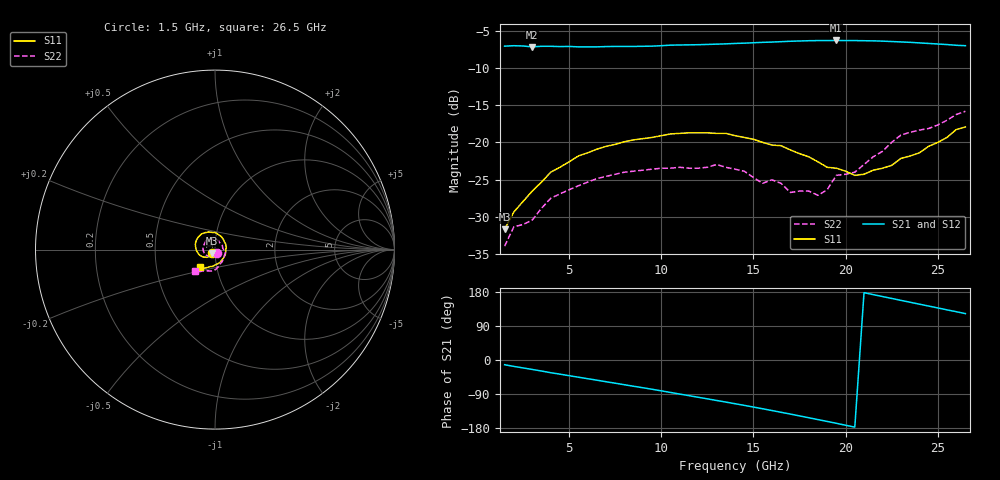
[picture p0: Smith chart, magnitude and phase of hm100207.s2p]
! HMMC-1002
! S-PARAMETERS at 7 dB attenuation setting. LAST UPDATED  07-06-99
# GHZ  S  MA  R  50
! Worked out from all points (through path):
!   51 points, 1.5 GHz to 26.5 GHz, reference 50 ohm
!   highest |S21| = -6.27 dB at 19.5 GHz (marker M1); lowest = -7.1 dB at 3 GHz (marker M2)
!   group delay of S21, straight-line fit = 24.9 ps
!   lowest |S11| = -31.7 dB at 1.5 GHz (marker M3), VSWR 1.05, Z = 48.2 - j1.82 ohm
!   |S11| at or under -10 dB: start of sweep to end of sweep
!   |S22| runs from -34.0 to -15.8 dB; largest |S21 - S12| = 0.0071
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1.5  0.026 -133.5  0.445 -12.5  0.442 -12.9  0.02 -62.8
2  0.034 -124.6  0.448 -16.9  0.446 -17.3  0.027 -70.5
3  0.047 -133.3  0.44 -24.9  0.441 -25.3  0.03 -103.0
4  0.063 -136.5  0.444 -33.5  0.443 -33.7  0.042 -108.9
6  0.085 -155.5  0.44 -49.3  0.44 -49.5  0.054 -139.9
8  0.101 -173.7  0.443 -65.3  0.442 -65.4  0.063 -161.9
10  0.111 169.1  0.448 -81.4  0.448 -81.5  0.067 175.9
13  0.115 136.8  0.459 -106.8  0.458 -106.8  0.071 136.1
14  0.111 124.4  0.464 -115.4  0.462 -115.3  0.066 124.2
15.5  0.1 103.6  0.472 -128.7  0.472 -128.7  0.053 93.2
16  0.096 97.8  0.474 -133.3  0.474 -133.2  0.056 81.7
16.5  0.095 90.0  0.477 -138.0  0.476 -137.9  0.053 66.5
17  0.089 81.1  0.48 -142.7  0.478 -142.6  0.046 60.4
18  0.08 63.5  0.484 -152.3  0.483 -152.2  0.047 29.2
18.5  0.074 51.2  0.485 -157.3  0.484 -157.1  0.044 10.0
19  0.068 40.1  0.485 -162.1  0.485 -161.9  0.048 0.3
19.5  0.067 26.9  0.486 -167.1  0.485 -166.9  0.06 -14.5
20.5  0.06 -0.2  0.485 -177.1  0.484 -176.9  0.063 -35.4
22.5  0.07 -58.1  0.478 162.5  0.477 162.9  0.1 -81.2
23  0.078 -69.5  0.475 157.4  0.473 157.8  0.112 -89.0
24.5  0.094 -97.9  0.464 142.4  0.463 142.8  0.124 -107.2
26.5  0.127 -130.6  0.448 122.4  0.447 123.3  0.162 -133.6
